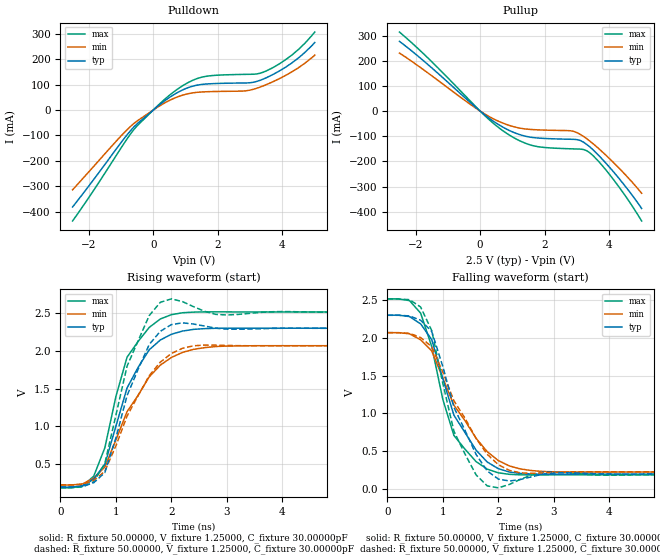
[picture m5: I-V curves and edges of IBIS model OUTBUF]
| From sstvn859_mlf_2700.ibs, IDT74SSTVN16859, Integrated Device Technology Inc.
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|   Model OUTBUF
[Model]   OUTBUF
Model_type   Output
Polarity   Inverting
Vmeas =  1.25000V
Cref = 30.00000pF
Rref =  50.00000
Vref =  1.25000V
C_comp   3.50000pF   3.50000pF   3.50000pF
[Temperature Range]   25.00000   70.00000   0.000
[Voltage Range]   2.50000V   2.30000V   2.70000V
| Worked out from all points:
|   slope of the pulldown table from 0 to 0.375 V, typ, clamps not added: 9.8 ohm
|   slope of the pullup table from 0 to 0.375 V, typ, clamps not added: 10.1 ohm
|   rising waveform, R_fixture 50.00000, V_fixture 1.25000, C_fixture 30.00000pF: 20-80 % time 636ps typ, 784ps min, 562ps max; typ from 0.197 V to 2.3 V
|   rising waveform, R_fixture 50.00000, V_fixture 1.25000, C_fixture 30.00000pF: 20-80 % time 574ps typ, 719ps min, 504ps max; typ from 0.199 V to 2.3 V
|   falling waveform, R_fixture 50.00000, V_fixture 1.25000, C_fixture 30.00000pF: 20-80 % time 673ps typ, 817ps min, 535ps max; typ from 2.3 V to 0.197 V
|   falling waveform, R_fixture 50.00000, V_fixture 1.25000, C_fixture 30.00000pF: 20-80 % time 609ps typ, 761ps min, 459ps max; typ from 2.3 V to 0.199 V
[Pulldown]
| voltage   I(typ)   I(min)   I(max)
-2.5V     -382.1mA   -314.5mA   -437.4mA
-1.1V     -145.6mA   -116.1mA   -169.6mA
-600mV    -66.63mA   -53.03mA   -76.8mA
100mV     10.92mA    8.522mA    12.56mA
600mV     57.64mA    43.69mA    68.13mA
1.1V      89.1mA     64.83mA    109.6mA
1.5V      100.7mA    71.03mA    129.3mA
2.9V      106.7mA    76.05mA    140.5mA
3.2V      112.5mA    85.58mA    142mA
3.5V      127.1mA    99.91mA    154mA
4.3V      186.2mA    151mA      217.4mA
5V        265.8mA    216.1mA    307.2mA
[Pullup]
| voltage   I(typ)   I(min)   I(max)
-2.5V     277.1mA    230.6mA    314.1mA
-1.5V     171.8mA    140.4mA    196.3mA
0V        -3.242nA   -2.817nA   -2.207nA
500mV     -48.16mA   -36.41mA   -58.24mA
900mV     -76.91mA   -56.88mA   -94.98mA
1.7V      -106mA     -74mA      -139.3mA
2.8V      -111.9mA   -78.26mA   -149.8mA
3.1V      -116.8mA   -92.51mA   -151mA
3.4V      -142.8mA   -119.5mA   -166.2mA
3.7V      -180mA     -152.3mA   -204.3mA
4.1V      -237mA     -200.8mA   -267.3mA
5V        -386.9mA   -326.4mA   -436.7mA
[Ramp]
| variable   typ   min   max
dV/dt_r   1.24620/0.15909n   1.08300/0.21706n   1.38720/0.12588n
dV/dt_f   1.25244/0.15723n   1.09230/0.21256n   1.38660/0.14172n
R_load = 50.00000
[Rising Waveform]
R_fixture = 50.00000
V_fixture = 1.25000
V_fixture_min = 1.15000
V_fixture_max = 1.35000
C_fixture = 30.00000pF
| time   V(typ)   V(min)   V(max)
0s        197.2mV    224.9mV    188mV
400ps     214.9mV    240.4mV    213.5mV
600ps     303.5mV    317.7mV    342.8mV
800ps     498.8mV    463.8mV    717.9mV
1ns       1.006V     823.8mV    1.398V
1.2ns     1.508V     1.195V     1.915V
1.6ns     2.014V     1.655V     2.309V
2ns       2.219V     1.912V     2.478V
3ns       2.298V     2.062V     2.514V
10ns      2.298V     2.067V     2.513V
[Rising Waveform]
R_fixture = 50.00000
V_fixture = 1.25000
V_fixture_min = 1.15000
V_fixture_max = 1.35000
C_fixture = 30.00000pF
R_dut = 0.11300
L_dut = 2.59000nH
C_dut = 0.19900pF
| time   V(typ)   V(min)   V(max)
0s        199.2mV    226.6mV    190.3mV
600ps     255.6mV    287.9mV    268.2mV
800ps     389.7mV    406.2mV    512.4mV
1ns       849.8mV    745.4mV    1.152V
1.2ns     1.407V     1.137V     1.796V
1.6ns     2.083V     1.671V     2.466V
1.8ns     2.257V     1.851V     2.641V
2.2ns     2.369V     2.033V     2.65V
2.6ns     2.326V     2.075V     2.521V
10ns      2.296V     2.066V     2.511V
[Falling Waveform]
R_fixture = 50.00000
V_fixture = 1.25000
V_fixture_min = 1.15000
V_fixture_max = 1.35000
C_fixture = 30.00000pF
| time   V(typ)   V(min)   V(max)
0s        2.298V     2.067V     2.513V
400ps     2.279V     2.051V     2.49V
600ps     2.182V     1.972V     2.324V
800ps     1.975V     1.825V     1.882V
1ns       1.457V     1.465V     1.184V
1.2ns     975.6mV    1.108V     707.7mV
1.6ns     513.5mV    670.2mV    362.2mV
2ns       268.9mV    376.1mV    214.7mV
3ns       196.4mV    227.9mV    187.5mV
10ns      197.2mV    224.9mV    188mV
[Falling Waveform]
R_fixture = 50.00000
V_fixture = 1.25000
V_fixture_min = 1.15000
V_fixture_max = 1.35000
C_fixture = 30.00000pF
R_dut = 0.11300
L_dut = 2.59000nH
C_dut = 0.19900pF
| time   V(typ)   V(min)   V(max)
0s        2.296V     2.066V     2.511V
400ps     2.288V     2.058V     2.502V
600ps     2.23V      2.002V     2.406V
800ps     2.083V     1.881V     2.094V
1.2ns     1.08V      1.165V     763.3mV
1.6ns     456.2mV    667.2mV    186.7mV
1.8ns     239.4mV    459mV      42.06mV
2.2ns     106.6mV    246.3mV    61.33mV
2.6ns     161.7mV    207.3mV    187mV
10ns      199.2mV    226.6mV    190.3mV
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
